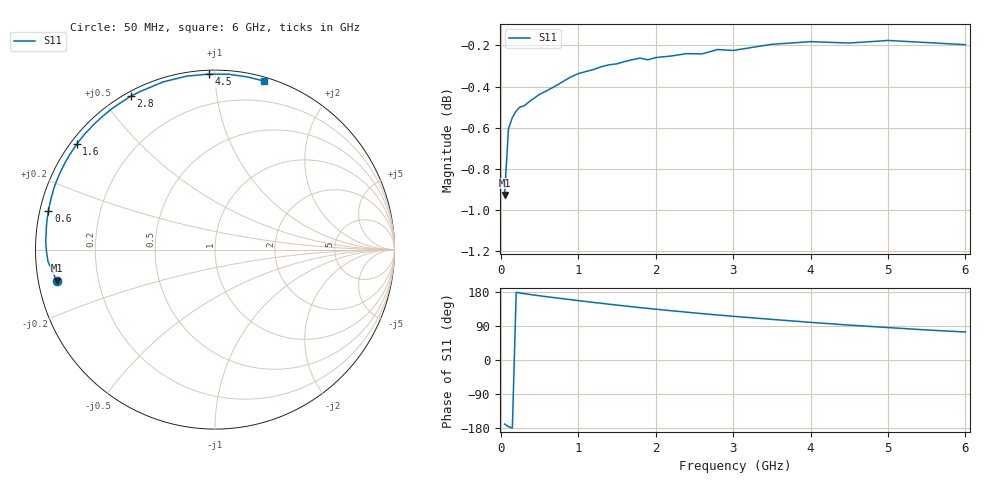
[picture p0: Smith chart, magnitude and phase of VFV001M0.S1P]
! Infineon Technologies  Discrete & RF Semiconductors
! BBY 58-03
! Si Tuning Diode in SOD323
! VR =
! S-Parameters:  June  1999
# GHz  S  MA  R  50
!  f  S11
! GHz  MAG  ANG
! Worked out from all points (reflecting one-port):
!   34 points, 50 MHz to 6 GHz, reference 50 ohm
!   lowest |S11| = -0.9 dB at 50 MHz (marker M1), VSWR 18.77, Z = 2.69 - j4.84 ohm
!   phase of S11 starts at -169 deg and turns -117 deg over the sweep
!   S11 on the Smith chart (normalised r, x): 50 MHz: 0.05, -0.10; 600 MHz: 0.02, +0.11; 1.6 GHz: 0.02, +0.34; 2.8 GHz: 0.02, +0.59; 4.5 GHz: 0.02, +0.96; 6 GHz: 0.03, +1.33
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0.05  0.8989 -168.9
0.1  0.9328 -175.9
0.15  0.9386 -179.2
0.2  0.9421 178.6
0.25  0.9442 176.8
0.4  0.948 172.2
0.5  0.9508 169.5
0.6  0.9529 166.9
0.8  0.9576 161.8
0.9  0.9601 159.3
1  0.9619 156.8
1.2  0.9642 151.9
1.3  0.9657 149.6
1.4  0.9667 147.2
1.6  0.9685 142.7
1.8  0.9703 138.2
2  0.9706 134.1
2.2  0.9715 130.0
2.4  0.9728 126.2
2.6  0.9726 122.4
2.8  0.975 118.8
3  0.9745 115.3
3.5  0.9779 107.2
4  0.9793 99.3
4.5  0.9786 92.1
5  0.98 85.6
5.5  0.9788 79.3
6  0.9777 73.9
